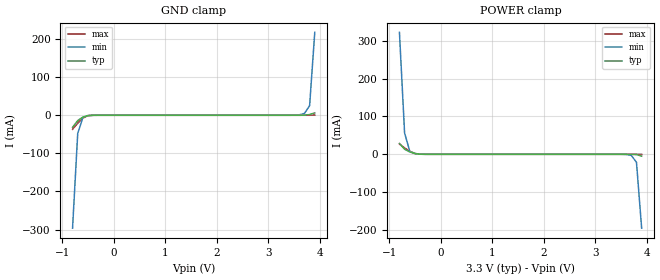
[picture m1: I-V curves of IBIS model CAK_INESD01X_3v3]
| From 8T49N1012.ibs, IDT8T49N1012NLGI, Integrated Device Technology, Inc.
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| 4.00000e+00   -1.39435e-02   -4.76170e-01   -2.47919e-03
| 4.10000e+00   -3.14988e-02   -7.57889e-01   -1.14633e-02
| 4.20000e+00   -2.28002e-01   -1.04024e+00   -2.64916e-02
| 4.30000e+00   -6.05524e-01   -1.32301e+00   -4.21848e-02
| 4.40000e+00   -9.83643e-01   -1.60614e+00   -8.92880e-02
| 4.50000e+00   -1.36229e+00   -1.88958e+00   -5.31426e-01
| 4.60000e+00   -1.74142e+00   -2.17332e+00   -1.01589e+00
| 4.70000e+00   -2.12097e+00   -2.45733e+00   -1.50090e+00
| 4.80000e+00   -2.50090e+00   -2.74162e+00   -1.98635e+00
| 4.90000e+00   -2.88116e+00   -3.02615e+00   -2.47218e+00
| 5.00000e+00   -3.26171e+00   -3.31092e+00   -2.95830e+00
| 5.10000e+00   -3.64251e+00   -3.59590e+00   -3.44467e+00
| 5.20000e+00   -4.02353e+00   -3.88109e+00   -3.93123e+00
| 5.30000e+00   -4.40474e+00   -4.16647e+00   -4.41796e+00
| 5.40000e+00   -4.78610e+00   -4.45202e+00   -4.90484e+00
| 5.50000e+00   -5.16760e+00   -4.73774e+00   -5.39184e+00
| 5.60000e+00   -5.54921e+00   -5.02360e+00   -5.87893e+00
| 5.70000e+00   -5.93093e+00   -5.30959e+00   -6.36610e+00
| 5.80000e+00   -6.31272e+00   -5.59572e+00   -6.85331e+00
| 5.90000e+00   -6.69459e+00   -5.88196e+00   -7.34056e+00
| 6.00000e+00   -7.07651e+00   -6.16831e+00   -7.82783e+00
| 6.10000e+00   -7.45848e+00   -6.45476e+00   -8.31510e+00
| 6.20000e+00   -7.84049e+00   -6.74131e+00   -8.80238e+00
| 6.30000e+00   -8.22253e+00   -7.02794e+00   -9.28965e+00
| 6.40000e+00   -8.60459e+00   -7.31465e+00   -9.77691e+00
| 6.50000e+00   -8.98667e+00   -7.60144e+00   -1.02642e+01
| 6.60000e+00   -9.36876e+00   -7.88830e+00   -1.07514e+01
[Model]   CAK_INESD01X_3v3
Model_type   Input
Polarity   Non-Inverting
Vinl = 0.8V
Vinh = 2.0V
|   typ   min   max
C_comp   13.5pF   12pF   15pF
|   typ   min   max
[Voltage range]   3.3V   3.135V   3.465V
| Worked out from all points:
|   GND clamp passes 1 mA (typ) near -0.51 V on its own axis
|   POWER clamp passes 1 mA (typ) near -0.45 V on its own axis
[GND_clamp]
|Voltage   I (typ)   I (min)   I (max)
|Note, modeling breaks down at 250mA and above.  This is well beyond the functional   |
|operating range of the device.  Should this scenario occur, catastrophic failure and   |
|possible damage to the device and/or board is of higher concern than the I-V curve   |
|behavior.  The IBIS checker will flag currents in excess of 10A with warnings.  Lines   |
|with currents in excess of 0.35 A have been commented out.  The points still remain|
|available to the user if the user desires to use them.   |
|-3.30000e+00   -9.36876e+00   -7.41789e+00   -1.15553e+01
|-3.20000e+00   -8.98667e+00   -7.13115e+00   -1.10681e+01
|-3.10000e+00   -8.60459e+00   -6.84449e+00   -1.05809e+01
|-3.00000e+00   -8.22253e+00   -6.55791e+00   -1.00936e+01
|-2.90000e+00   -7.84049e+00   -6.27142e+00   -9.60637e+00
|-2.80000e+00   -7.45848e+00   -5.98504e+00   -9.11911e+00
|-2.70000e+00   -7.07651e+00   -5.69875e+00   -8.63183e+00
|-2.60000e+00   -6.69459e+00   -5.41259e+00   -8.14455e+00
|-2.50000e+00   -6.31272e+00   -5.12654e+00   -7.65728e+00
|-2.40000e+00   -5.93093e+00   -4.84063e+00   -7.17002e+00
|-2.30000e+00   -5.54921e+00   -4.55486e+00   -6.68278e+00
|-2.20000e+00   -5.16760e+00   -4.26925e+00   -6.19558e+00
|-2.10000e+00   -4.78610e+00   -3.98381e+00   -5.70844e+00
|-2.00000e+00   -4.40474e+00   -3.69855e+00   -5.22138e+00
|-1.90000e+00   -4.02353e+00   -3.41349e+00   -4.73442e+00
|-1.80000e+00   -3.64251e+00   -3.12864e+00   -4.24759e+00
|-1.70000e+00   -3.26171e+00   -2.84402e+00   -3.76091e+00
|-1.60000e+00   -2.88116e+00   -2.55965e+00   -3.27441e+00
|-1.50000e+00   -2.50090e+00   -2.27553e+00   -2.78813e+00
|-1.40000e+00   -2.12097e+00   -1.99169e+00   -2.30210e+00
|-1.30000e+00   -1.74142e+00   -1.70814e+00   -1.81640e+00
|-1.20000e+00   -1.36229e+00   -1.42490e+00   -1.33109e+00
|-1.10000e+00   -9.83643e-01   -1.14199e+00   -8.46264e-01
|-1.00000e+00   -6.05524e-01   -8.59476e-01   -3.62007e-01
|-9.00000e-01   -2.28002e-01   -5.77494e-01   -5.70861e-02
-800mV    -31.5mA    -296.3mA   -37.03mA
-700mV    -13.94mA   -47.89mA   -20.77mA
-600mV    -4.814mA   -5.925mA   -7.477mA
-500mV    -769.5uA   -876.2uA   -1.11mA
-400mV    -50.39uA   -91.12uA   -52.98uA
3.4V      929.4pA    7.738uA    18.23pA
3.6V      7.536uA    1.177mA    576.1pA
3.7V      200.6uA    4.949mA    206.1nA
3.8V      1.845mA    25.21mA    18.18uA
3.9V      6.193mA    217.6mA    563.4uA
| 4.00000e+00   1.34293e-02   5.06540e-01   3.84286e-03
| 4.10000e+00   2.85679e-02   7.94900e-01   1.06020e-02
| 4.20000e+00   2.42102e-01   1.08355e+00   2.05441e-02
| 4.30000e+00   6.27135e-01   1.37257e+00   3.02103e-02
| 4.40000e+00   1.01263e+00   1.66196e+00   7.70913e-02
| 4.50000e+00   1.39863e+00   1.95172e+00   5.37431e-01
| 4.60000e+00   1.78513e+00   2.24185e+00   1.03062e+00
| 4.70000e+00   2.17212e+00   2.53235e+00   1.52443e+00
| 4.80000e+00   2.55958e+00   2.82322e+00   2.01885e+00
| 4.90000e+00   2.94751e+00   3.11446e+00   2.51386e+00
| 5.00000e+00   3.33588e+00   3.40606e+00   3.00943e+00
| 5.10000e+00   3.72470e+00   3.69803e+00   3.50553e+00
| 5.20000e+00   4.11396e+00   3.99038e+00   4.00216e+00
| 5.30000e+00   4.50363e+00   4.28310e+00   4.49928e+00
| 5.40000e+00   4.89373e+00   4.57620e+00   4.99688e+00
| 5.50000e+00   5.28425e+00   4.86969e+00   5.49495e+00
| 5.60000e+00   5.67518e+00   5.16358e+00   5.99346e+00
| 5.70000e+00   6.06653e+00   5.45787e+00   6.49241e+00
| 5.80000e+00   6.45829e+00   5.75259e+00   6.99179e+00
| 5.90000e+00   6.85048e+00   6.04774e+00   7.49160e+00
| 6.00000e+00   7.24309e+00   6.34335e+00   7.99183e+00
| 6.10000e+00   7.63615e+00   6.63943e+00   8.49248e+00
| 6.20000e+00   8.02966e+00   6.93599e+00   8.99355e+00
| 6.30000e+00   8.42363e+00   7.23307e+00   9.49506e+00
| 6.40000e+00   8.81808e+00   7.53069e+00   9.99700e+00
| 6.50000e+00   9.21303e+00   7.82887e+00   1.04994e+01
| 6.60000e+00   9.60850e+00   8.12763e+00   1.10022e+01
[Power_clamp]
|Voltage   I (typ)   I (min)   I (max)
|Note, modeling breaks down at 250mA and above.  This is well beyond the functional   |
|operating range of the device.  Should this scenario occur, catastrophic failure and   |
|possible damage to the device and/or board is of higher concern than the I-V curve   |
|behavior.  The IBIS checker will flag currents in excess of 10A with warnings.  Lines   |
|with currents in excess of 0.35 A have been commented out.  The points still remain|
|available to the user if the user desires to use them.   |
|-3.30000e+00   9.60850e+00   7.63797e+00   1.18330e+01
|-3.20000e+00   9.21303e+00   7.34015e+00   1.13293e+01
|-3.10000e+00   8.81808e+00   7.04288e+00   1.08262e+01
|-3.00000e+00   8.42363e+00   6.74613e+00   1.03235e+01
|-2.90000e+00   8.02966e+00   6.44988e+00   9.82127e+00
|-2.80000e+00   7.63615e+00   6.15411e+00   9.31948e+00
|-2.70000e+00   7.24309e+00   5.85879e+00   8.81813e+00
|-2.60000e+00   6.85048e+00   5.56392e+00   8.31720e+00
|-2.50000e+00   6.45829e+00   5.26948e+00   7.81670e+00
|-2.40000e+00   6.06653e+00   4.97544e+00   7.31662e+00
|-2.30000e+00   5.67518e+00   4.68181e+00   6.81696e+00
|-2.20000e+00   5.28425e+00   4.38857e+00   6.31773e+00
|-2.10000e+00   4.89373e+00   4.09571e+00   5.81893e+00
|-2.00000e+00   4.50363e+00   3.80323e+00   5.32057e+00
|-1.90000e+00   4.11396e+00   3.51113e+00   4.82267e+00
|-1.80000e+00   3.72470e+00   3.21939e+00   4.32523e+00
|-1.70000e+00   3.33588e+00   2.92802e+00   3.82828e+00
|-1.60000e+00   2.94751e+00   2.63702e+00   3.33184e+00
|-1.50000e+00   2.55958e+00   2.34639e+00   2.83591e+00
|-1.40000e+00   2.17212e+00   2.05612e+00   2.34054e+00
|-1.30000e+00   1.78513e+00   1.76623e+00   1.84573e+00
|-1.20000e+00   1.39863e+00   1.47670e+00   1.35152e+00
|-1.10000e+00   1.01263e+00   1.18756e+00   8.57930e-01
|-1.00000e+00   6.27135e-01   8.98775e-01   3.64964e-01
|-9.00000e-01   2.42102e-01   6.10330e-01   4.20775e-02
-800mV    28.57mA    321.9mA    27.12mA
-700mV    13.43mA    56.36mA    16.78mA
-600mV    6.193mA    8.187mA    7.847mA
-500mV    1.845mA    2.071mA    2.293mA
-300mV    7.536uA    23.16uA    4.595uA
3.5V      -38.15nA   -37.11uA   -1.389nA
3.7V      -50.39uA   -3.041mA   -40.99nA
3.8V      -769.5uA   -21.19mA   -4.022uA
3.9V      -4.814mA   -194.9mA   -172.8uA
